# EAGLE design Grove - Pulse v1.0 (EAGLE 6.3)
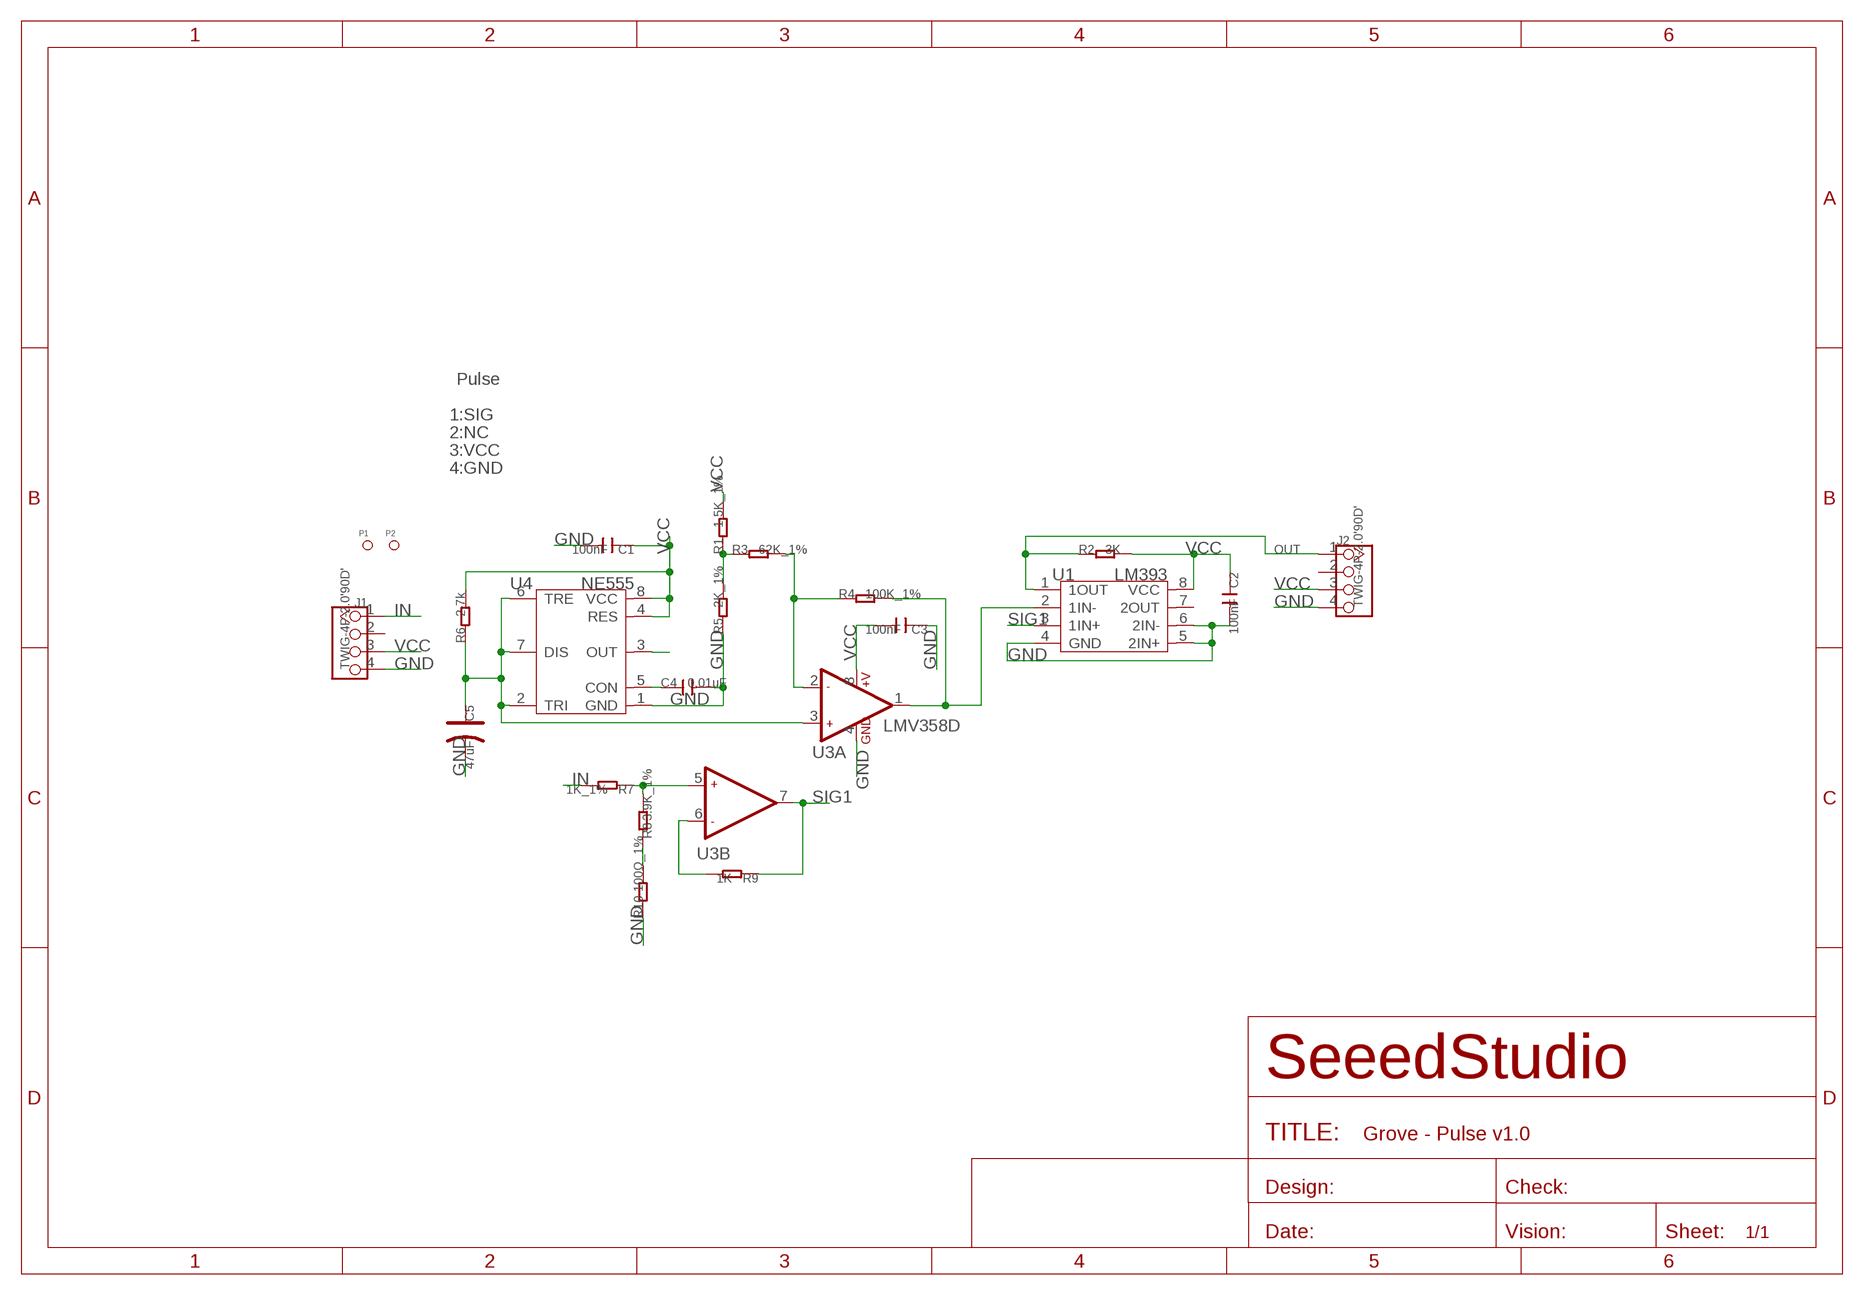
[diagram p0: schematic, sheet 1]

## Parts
C1  100nF  C-0603  [C0603]
C2  100nF  C-0603  [C0603]
C3  100nF  C-0603  [C0603]
C4  0.01uF  C-0603  [C0603]
C5  47uF  CAP-AVX-B  [AVX-B]
J1  TWIG-4P-2.0'90D'  [4P-2.0-90D]
J2  TWIG-4P-2.0'90D'  [4P-2.0-90D]
P1  PAD-MARK  [ROUND-MARK-1.0]
P2  PAD-MARK  [ROUND-MARK-1.0]
R1  1.5K_1%  R-0603  [R0603]
R2  3K  R-0603  [R0603]
R3  62K_1%  R-0603  [R0603]
R4  100K_1%  R-0603  [R0603]
R5  2K_1%  R-0603  [R0603]
R6  2.7k  R-0603  [R0603]
R7  1K_1%  R-0603  [R0603]
R8  3.9K_1%  R-0603  [R0603]
R9  1K  R-0603  [R0603]
R10  100Ω_1%  R-0603  [R0603]
U1  LM393  LM293D  [SOIC8-6.0]
U3  LMV358D  [SO08]
U4  NE555  NE555'TS555IPT'  [TSSOP8]

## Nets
GND: C1.2 C2.2 C3.1 C4.2 C5.- J1.4 J2.4 R5.1 R10.1 U1.4(GND) U1.5(2IN+) U1.6(2IN-) U3.4(A:GND) U4.1(GND)
IN: J1.1 R7.2
N$1: U4.3(OUT)
N$8: C5.+ R6.1 U3.3(A:+IN1) U4.2(TRI) U4.6(TRE) U4.7(DIS)
N$10: C4.1 U4.5(CON)
N$13: R3.2 R4.1 U3.2(A:-IN1)
N$14: R4.2 U1.2(1IN-) U3.1(A:OUT1)
N$15: R1.1 R3.1 R5.2
N$16: R7.1 R8.2 U3.5(B:+IN2)
N$17: R8.1 R10.2
N$18: R9.2 U3.6(B:-IN2)
OUT: J2.1 R2.1 U1.1(1OUT)
SIG1: R9.1 U1.3(1IN+) U3.7(B:OUT2)
VCC: C1.1 C2.1 C3.2 J1.3 J2.3 R1.2 R2.2 R6.2 U1.8(VCC) U3.8(A:+V) U4.4(RES) U4.8(VCC)
Unconnected: J1.2 J2.2 U1.7(2OUT)

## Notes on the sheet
- Pulse
- 1:SIG
- 2:NC
- 3:VCC
- 4:GND

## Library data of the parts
C1-C4 = Discrete:C*: Ceramic Capacitors
C5 = Discrete:CAP*: Electrolytic Capacitors,Tantalum Capacitors and Super Capacitors
J1 J2 = Connector:TWIG-4P-2.0
P1 P2 = Discrete:PAD-MARK; PARTNO: DNP
R1-R10 = Discrete:R*
U1 = template:LM293: Dual Differential Comparator
U3 = IC:LMV358: General purpose LOW Voltage, Rail-to-Rail Output Amplifiers http://www.fairchildsemi.com/ds/LM/LMV358.pdf
U4 = IC:NE555: General Purpose Single Bipolar Timers

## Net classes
0 default: width 0.152 mm, drill 0.305 mm, clearance 0.152 mm

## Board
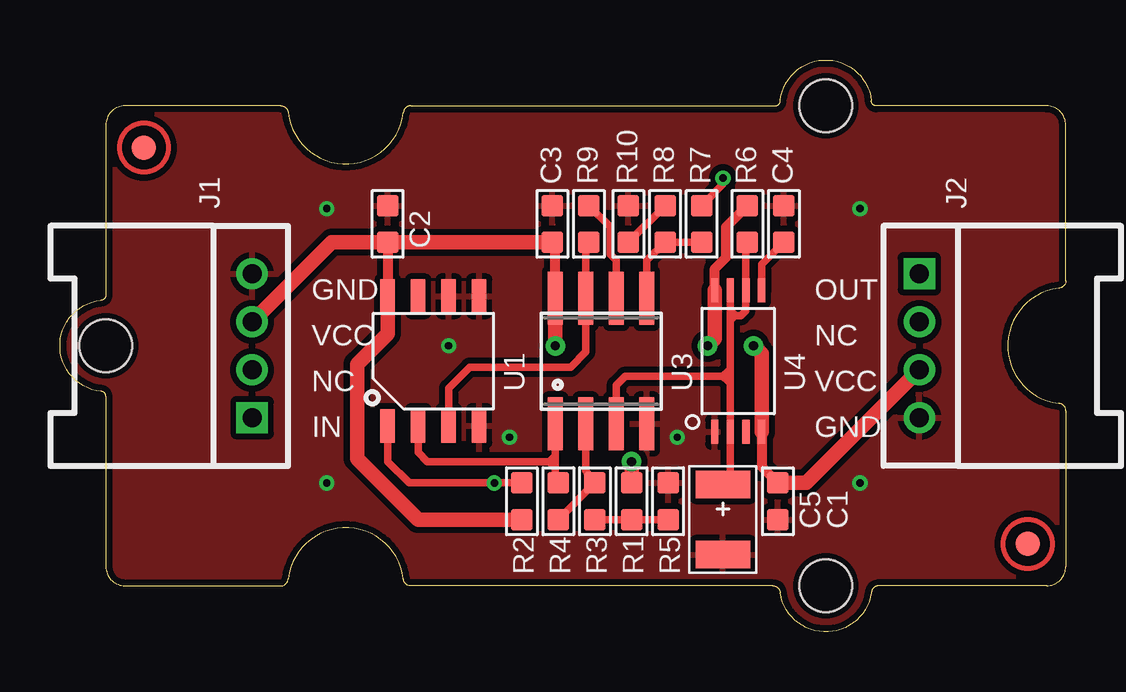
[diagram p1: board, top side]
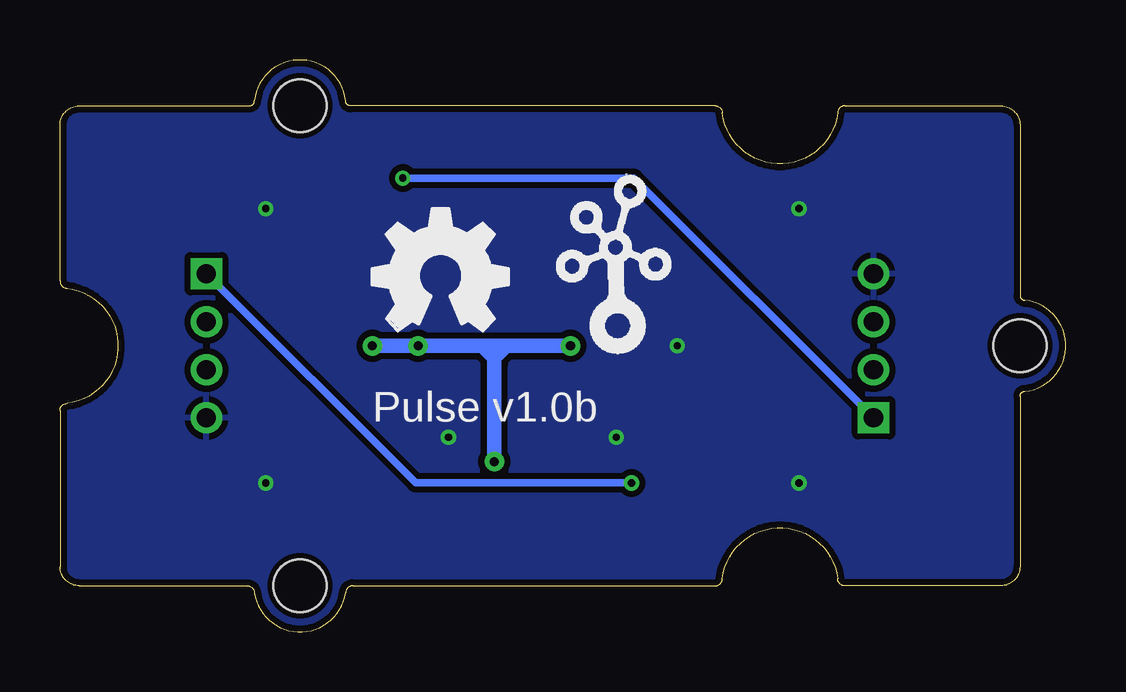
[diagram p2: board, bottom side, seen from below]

Size 41.91 x 23.83 mm. Coordinates in mm from the lower left corner, seen from the top.
Copper layers (1*16): Top 0.035mm / dielectric 1.5mm / Bottom 0.035mm
Design rules "default": minimum track width 6mil, minimum drill 12mil, track to track 6mil, track to pad 6mil, pad to pad 6mil, via to via 6mil, smd to smd 0mil, copper to edge 10mil, drill to drill 10mil, minimum pad ring 10mil, minimum via ring 6mil, stop-mask expansion 2mil, vias tented up to drill 100mil, thermal gap 10mil

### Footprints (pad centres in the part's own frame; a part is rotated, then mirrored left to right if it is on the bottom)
C0603 = smd 0.889 x 0.889: 1 -0.762,0; 2 0.762,0
AVX-B = smd 1.143 x 2.286: + -1.46,0; - 1.46,0
4P-2.0-90D = drill 0.8 pad 1.27 square: 1 -3,0 | drill 0.8 pad 1.27: 2 -1,0; 3 1,0; 4 3,0
ROUND-MARK-1.0 = smd 1.016 x 1.016: P$1 0,0
R0603 = smd 0.889 x 0.889: 1 -0.762,0; 2 0.762,0
SOIC8-6.0 = smd 0.6 x 1.4: 1 -1.905,-2.7; 2 -0.635,-2.7; 3 0.635,-2.7; 4 1.905,-2.7; 5 1.905,2.7; 6 0.635,2.7; 7 -0.635,2.7; 8 -1.905,2.7
SO08 = smd 0.61 x 2.21: 1 -1.905,-2.616; 2 -0.635,-2.616; 3 0.635,-2.616; 4 1.905,-2.616; 5 1.905,2.616; 6 0.635,2.616; 7 -0.635,2.616; 8 -1.905,2.616
TSSOP8 = smd 0.3 x 1: 1 -0.975,-2.95; 2 -0.325,-2.95; 3 0.325,-2.95; 4 0.975,-2.95; 5 0.975,2.95; 6 0.325,2.95; 7 -0.325,2.95; 8 -0.975,2.95
2U-DIM-W/DRILL = hole 2.2: -10,-10; -10,10; 20,0

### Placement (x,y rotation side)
C1  29.91,5.44 270 top
C2  13.65,17 90 top
C3  20.51,17 270 top
C4  30.16,17 90 top
C5  27.62,4.68 270 top
J1  8.01,11.92 90 top
J2  35.81,11.92 270 top
P1  3.49,20.18 0 top
P2  40.32,3.67 0 top
R1  23.81,5.44 90 top
R2  19.24,5.44 270 top
R3  22.29,5.44 90 top
R4  20.77,5.44 90 top
R5  25.34,5.44 270 top
R6  28.64,17 90 top
R7  26.73,17 90 top
R8  25.21,17 270 top
R9  22.04,17 90 top
R10  23.69,17 270 top
U1  15.56,11.29 0 top
U3  22.54,11.29 0 top
U4  28.26,11.29 0 top
U$1  [2U-DIM-W/DRILL]  21.91,11.92 180 top
U$2  [OSHW_FILLX200_NOTEXT]  28.89,12.56 0 bottom
U$3  [TWIGLOGO]  18.73,12.56 0 bottom

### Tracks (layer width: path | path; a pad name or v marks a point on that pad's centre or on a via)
GND  (via drill 0.3 pad 0.64)
  other vias: 16.19,11.92 18.73,8.11 25.72,8.11 11.11,6.21 11.11,17.64 33.34,6.21 33.34,17.64
  pour Bottom (isolate 0.254): 42.23,-0.14 -0.32,-0.14 -0.32,23.99 42.23,23.99
  pour Top (isolate 0.254): 42.23,-0.14 -0.32,-0.14 -0.32,23.99 42.23,23.99
IN  (via drill 0.3 pad 0.64)
  Top 0.305: v27.62,18.91 27.62,18.65 R7.2
  Bottom 0.305: v27.62,18.91 17.99,18.91 J1.1
N$8
  Top 0.305: 27.93,10.65 U4.2 27.93,6.58 C5.+ | 27.93,10.65 27.93,12.99 | 27.93,12.99 27.93,13.17 | 27.93,13.17 U4.7 | 27.93,13.17 28.16,13.17 | 28.16,13.17 28.36,13.17 28.58,13.39 U4.6 28.58,16.18 R6.1 | 28.16,13.17 | 28.16,13.17 28.13,13.19 | 28.13,13.19 28,13.32 | 27.93,12.99 28.13,13.19 | U3.3 23.18,10.27 23.56,10.65 27.62,10.65 | 27.62,10.65 27.93,10.65 | 27.88,10.91 27.62,10.65 | 27.62,10.65 27.88,10.4
N$10
  Top 0.305: U4.5 29.23,15.31 C4.1
N$13
  Top 0.305: U3.2 21.91,6.71 R3.2 R4.1
N$14
  Top 0.305: U3.1 20.64,7.35 | 20.64,7.35 20.64,7.1 | 20.64,7.1 20.64,6.84 | 20.64,6.84 20.64,6.46 R4.2 | U1.2 14.92,7.48 15.3,7.1 20.38,7.1 | 20.38,7.1 20.64,7.1 | 20.64,6.84 20.38,7.1 | 20.38,7.1 20.64,7.35
N$15
  Top 0.305: R3.1 R1.1 R5.2
N$16
  Top 0.305: R7.1 R8.2 24.45,15.48 U3.5
N$17
  Top 0.305: R8.1 R10.2
N$18
  Top 0.305: U3.6 23.18,15.48 22.92,15.73 22.92,16.87 R9.2
OUT  (via drill 0.3 pad 0.64)
  Top 0.305: R2.1 19.11,6.21 v18.1,6.21 14.54,6.21 13.65,7.1 U1.1
  Bottom 0.305: v18.1,6.21 27.09,6.21 J2.1
SIG1
  Top 0.305: R9.1 21.91,16.11 U3.7 21.91,11.67 21.27,11.03 17.08,11.03 16.19,10.14 U1.3
VCC  (via drill 0.38 pad 0.81)
  Top 0.406: C2.1 U1.8 | U3.8 20.64,16.11 C3.2 | U4.4 29.23,6.88 C1.1 | R6.2 27.75,16.87 27.75,15.6 27.28,15.14 U4.8
  Top 0.61: U1.8 13.65,12.43 12.38,11.16 12.38,7.22 14.92,4.68 R2.2 | R1.2 v23.81,7.1 | C1.1 31.09,6.21 J2.3 | J1.3 11.33,16.24 C2.1 C3.2 | U4.4 29.23,11.58 v28.89,11.92 | U4.8 27.28,12.22 v26.99,11.92 | U3.8 v20.64,11.92
  Bottom 0.61: 23.94,11.92 v26.99,11.92 v28.89,11.92 | 23.94,11.92 v20.64,11.92 | v23.81,7.1 23.81,11.16 23.81,11.41 | 23.81,11.41 23.81,11.79 23.94,11.92 | 23.81,11.41 23.43,11.79 | 23.81,11.41 24.19,11.79

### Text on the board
tPlace: GND | OUT | VCC | NC | NC | VCC | IN | GND
bPlace: Pulse v1.0b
